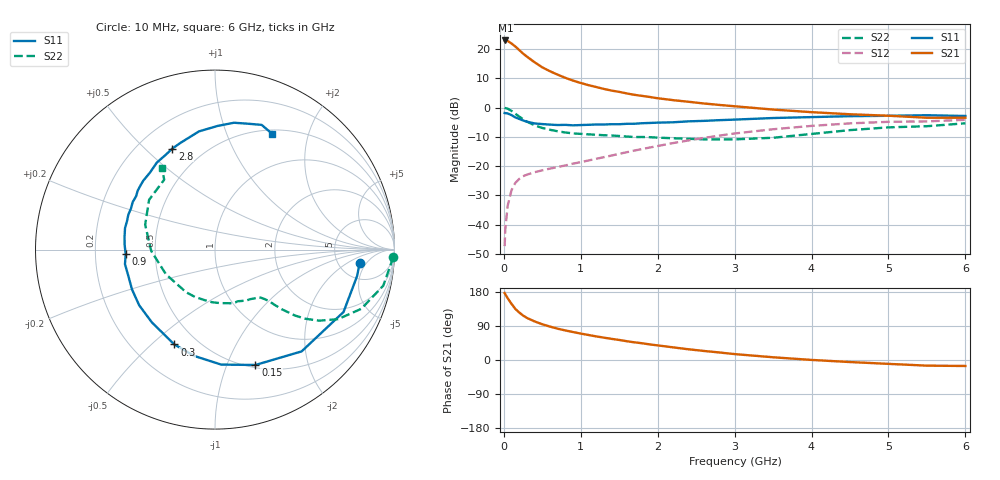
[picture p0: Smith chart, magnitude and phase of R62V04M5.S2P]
! SIEMENS Small Signal Semiconductors
! BFR193
! Si NPN RF Bipolar Junction Transistor in SOT23
! VCE = 2 V  IC = 4.5 mA
! Common Emitter S-Parameters:  May  1996
# GHz  S  MA  R  50
!  f  S11  S21  S12  S22
! GHz  MAG  ANG  MAG  ANG  MAG  ANG  MAG  ANG
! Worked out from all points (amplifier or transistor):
!   36 points, 10 MHz to 6 GHz, reference 50 ohm
!   highest |S21| = 23.0 dB at 20 MHz (marker M1)
!   |S21| within 3 dB of that: start of sweep to 188.4 MHz
!   unconditionally stable (mu >= 1): 896.7 MHz to 2.03 GHz
!   at 250 MHz: K = 0.40, MSG = 20.9 dB, |S12| = -23.4 dB
!   at 1.4 GHz: K = 1.07, MAG = 9.5 dB, |S12| = -16.4 dB
!   at 6 GHz: K = 0.98, MSG = 0.4 dB, |S12| = -4.2 dB
!   S11 on the Smith chart (normalised r, x): 10 MHz: 7.98, -3.46; 150 MHz: 0.53, -1.27; 300 MHz: 0.38, -0.59; 900 MHz: 0.33, -0.02; 2.8 GHz: 0.34, +0.61; 6 GHz: 0.54, +1.46
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0.01  0.8095 -5.3  13.91 176.8  0.0043 86.2  0.9926 -2.4
0.02  0.8054 -10.5  14.05 173.0  0.0087 82.4  0.9825 -4.9
0.05  0.796 -25.9  13.75 163.1  0.0212 76.4  0.9589 -12.1
0.1  0.7447 -49.6  12.44 148.1  0.0391 66.5  0.8796 -22.0
0.15  0.6811 -70.7  11.06 134.7  0.052 58.1  0.7871 -29.5
0.2  0.6416 -86.9  9.631 125.3  0.0606 52.7  0.7027 -34.3
0.25  0.6038 -100.9  8.374 117.4  0.0673 49.0  0.6345 -37.4
0.3  0.5751 -113.2  7.434 111.0  0.0716 46.7  0.5777 -39.5
0.4  0.5368 -130.9  5.953 101.8  0.0789 45.0  0.4976 -41.8
0.5  0.5241 -143.7  4.877 94.3  0.0849 44.8  0.4495 -42.9
0.6  0.5129 -154.4  4.181 88.1  0.0909 45.8  0.4184 -43.6
0.7  0.5046 -163.4  3.656 82.6  0.0968 47.5  0.3942 -44.7
0.9  0.4984 -177.0  2.894 73.8  0.1106 50.8  0.363 -47.1
1.1  0.5092 171.8  2.423 66.0  0.1251 53.6  0.35 -50.9
1.3  0.5151 162.3  2.09 59.0  0.1426 55.7  0.3378 -55.0
1.6  0.5295 149.9  1.746 49.5  0.1733 57.7  0.3207 -63.3
2.2  0.562 130.0  1.342 33.4  0.2481 56.4  0.2998 -84.1
2.8  0.6108 112.9  1.113 19.9  0.3324 50.3  0.2864 -112.9
3.5  0.6647 97.7  0.927 7.2  0.4274 39.3  0.3057 -153.0
4.5  0.7147 81.5  0.771 -5.4  0.5388 22.2  0.4131 160.4
5.5  0.7419 69.5  0.672 -14.9  0.5826 5.0  0.4816 126.0
6  0.7199 63.9  0.673 -15.8  0.6196 0.1  0.5407 123.1
